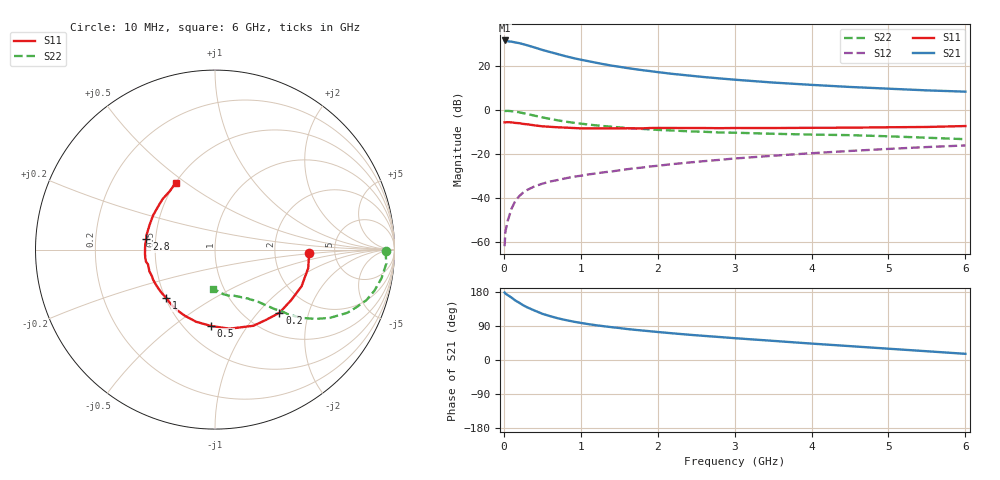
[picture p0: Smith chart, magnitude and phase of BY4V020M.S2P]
! SIEMENS Small Signal Semiconductors
! BFY420
! Si NPN RF SIEGET Grounded Emitter Transistor in MICRO-X
! VCE = 4 V  IC = 20 mA
! Common Emitter S-Parameters:  October  1996
# GHz  S  MA  R  50
!  f  S11  S21  S12  S22
! GHz  MAG  ANG  MAG  ANG  MAG  ANG  MAG  ANG
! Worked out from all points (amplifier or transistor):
!   36 points, 10 MHz to 6 GHz, reference 50 ohm
!   highest |S21| = 31.7 dB at 10 MHz (marker M1)
!   |S21| within 3 dB of that: start of sweep to 380.9 MHz
!   unconditionally stable (mu >= 1): start of sweep to 15.24 MHz; 1.998 GHz to end of sweep
!   at 250 MHz: K = 0.34, MSG = 33.8 dB, |S12| = -37.6 dB
!   at 1.4 GHz: K = 0.91, MSG = 24.1 dB, |S12| = -28.0 dB
!   at 6 GHz: K = 1.06, MAG = 10.7 dB, |S12| = -16.1 dB
!   S11 on the Smith chart (normalised r, x): 10 MHz: 3.19, -0.17; 200 MHz: 1.40, -1.32; 500 MHz: 0.67, -0.70; 1 GHz: 0.50, -0.32; 2.8 GHz: 0.44, +0.06; 6 GHz: 0.50, +0.46
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0.01  0.5233 -2.1  38.28 178.0  0.0008 49.6  0.9529 -0.4
0.02  0.5247 -4.2  37.84 175.4  0.0017 59.9  0.9508 -1.4
0.05  0.5294 -11.3  36.64 171.3  0.003 71.4  0.958 -4.6
0.1  0.5238 -23.0  35.88 164.7  0.0057 76.8  0.9416 -9.7
0.15  0.5092 -33.6  34.49 156.9  0.0086 72.1  0.9175 -14.4
0.2  0.5029 -44.4  33.26 151.1  0.011 71.0  0.8891 -18.5
0.25  0.4837 -54.2  31.59 144.7  0.0132 66.6  0.8505 -22.2
0.3  0.4751 -63.3  29.85 139.3  0.0151 66.0  0.8174 -25.5
0.4  0.4481 -79.6  26.49 130.4  0.0184 63.1  0.745 -30.7
0.5  0.4262 -92.8  23.35 122.0  0.0211 61.6  0.6818 -34.5
0.6  0.4157 -104.6  20.88 115.8  0.0236 59.8  0.6282 -37.4
0.7  0.4054 -114.1  18.75 110.2  0.0256 59.6  0.5841 -39.6
0.8  0.3983 -122.5  16.82 105.6  0.0279 58.2  0.5465 -41.4
1  0.3827 -135.3  13.96 97.9  0.032 59.2  0.4907 -43.7
1.1  0.3832 -141.0  12.92 94.6  0.0343 58.6  0.4677 -45.0
1.6  0.3849 -161.6  9.036 81.8  0.045 58.9  0.3898 -49.5
2.2  0.3908 -176.5  6.628 70.3  0.0591 57.9  0.3421 -54.5
2.8  0.3871 171.3  5.252 60.7  0.0735 55.4  0.309 -59.1
3.5  0.3896 159.2  4.222 50.5  0.0913 51.3  0.2885 -64.5
4.5  0.3971 143.6  3.35 36.6  0.1173 43.9  0.2684 -73.0
5.5  0.412 127.5  2.8 23.1  0.144 35.3  0.2345 -85.1
6  0.4326 120.3  2.619 16.3  0.1566 30.6  0.2172 -93.0
